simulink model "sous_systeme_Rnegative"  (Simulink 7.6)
settings: Solver=ode45  StartTime=0.0  StopTime=10.0  RelTol=1e-3
libraries: fl_lib x4, elec_lib x1

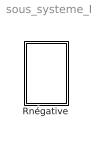
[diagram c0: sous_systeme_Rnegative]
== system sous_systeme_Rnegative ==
  Rnégative : Subsystem

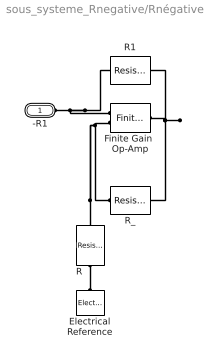
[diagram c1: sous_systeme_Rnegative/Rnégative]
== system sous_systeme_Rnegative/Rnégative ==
  Electrical Reference : fl_lib/Electrical/Electrical Elements/Electrical Reference  DialogController=NetworkEngine.DynNeDlgSource  SystemSampleTime=-1  i_Log=off  LocalVarNames=|i  LocalVarDescs=|i  LocalVarLogging=0
  Finite Gain  Op-Amp : elec_lib/Integrated Circuits/Finite Gain Op-Amp  DialogController=NetworkEngine.DynNeDlgSource  SystemSampleTime=-1  A=1000  Rin=1e+6 Ohm  Rout=100 Ohm  Vmin=-15 V  Vmax=15 V  LocalVarLogging=[]
  R : fl_lib/Electrical/Electrical Elements/Resistor  DialogController=NetworkEngine.DynNeDlgSource  SystemSampleTime=-1  R=1 kOhm  i_Log=off  v_Log=off  LocalVarNames=|i|v  LocalVarDescs=|i|v  LocalVarLogging=[0 0]
  R1 : fl_lib/Electrical/Electrical Elements/Resistor  DialogController=NetworkEngine.DynNeDlgSource  SystemSampleTime=-1  R=1 kOhm  i_Log=off  v_Log=off  LocalVarNames=|i|v  LocalVarDescs=|i|v  LocalVarLogging=[0 0]
  R_ : fl_lib/Electrical/Electrical Elements/Resistor  DialogController=NetworkEngine.DynNeDlgSource  SystemSampleTime=-1  R=1 kOhm  i_Log=off  v_Log=off  LocalVarNames=|i|v  LocalVarDescs=|i|v  LocalVarLogging=[0 0]
  -R1 : PMIOPort  Port=1  Side=Left
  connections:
  R/RConn1 -- Electrical Reference/LConn1
  -R1/RConn1 -- R1/LConn1 -- Finite Gain  Op-Amp/LConn1
  Finite Gain  Op-Amp/LConn2 -- R/LConn1 -- R_/LConn1
  Finite Gain  Op-Amp/RConn1 -- R1/RConn1 -- R_/RConn1
